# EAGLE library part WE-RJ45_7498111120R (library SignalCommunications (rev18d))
Order Code 7498111120R Design SMD xBase-T 10/100/1000 Base-T Ports 1x1 Application Standard Tab Position UP LED (Left-Right) YELLOW-GREEN EMI Fingers Yes Details see: http://katalog.we-online.de/en/pbs/WE-LAN_RJ45/7498111120R? Updated by Yingchun Shan 2016-08-23 2014 (C) Würth Elektronik
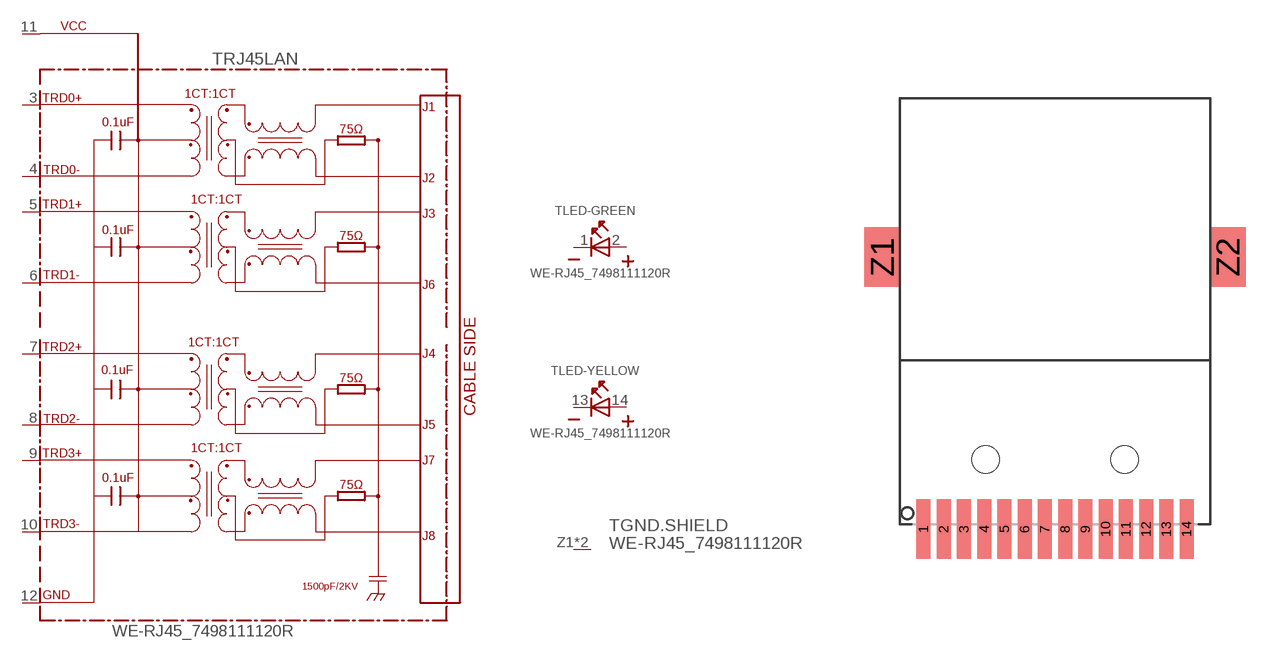
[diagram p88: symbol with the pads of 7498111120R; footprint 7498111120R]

Designator prefix T; gates RJ45LAN=7498111120R LED-GREEN=LED2PIN LED-YELLOW=LED2PIN GND.SHIELD=GNDPIN

## WE-RJ45_7498111120R (COMPANY-URL: http://www.we-online.de; CREATED-BY: Christin Zierenner; CREATED-DATE: AUG 2012; DATASHEET-URL: http://katalog.we-online.de/kataloge/eisos/media/pdf/7498111120R.pdf; MANUFACTURER: Würth Elektronik eiSos GmbH)  [7498111120R]
1  LED-GREEN:K  pas
2  LED-GREEN:A  pas
3  RJ45LAN:TRD0+
4  RJ45LAN:TRD0-
5  RJ45LAN:TRD1+
6  RJ45LAN:TRD1-
7  RJ45LAN:TRD2+
8  RJ45LAN:TRD2-
9  RJ45LAN:TRD3+
10  RJ45LAN:TRD3-
11  RJ45LAN:VCC  pwr
12  RJ45LAN:GND  pwr
13  LED-YELLOW:K  pas
14  LED-YELLOW:A  pas
Z1  GND.SHIELD:GND  pwr
Z2  GND.SHIELD:GND  pwr

## Footprint 7498111120R (pad centres in mm)
MAX HEIGHT=11.30mm PORTS----1X1 LED --Yes
smd 0.71 x 3: 1 -6.63,-3.5; 2 -5.61,-3.5; 3 -4.59,-3.5; 4 -3.57,-3.5; 5 -2.55,-3.5; 6 -1.53,-3.5; 7 -0.51,-3.5; 8 0.51,-3.5; 9 1.53,-3.5; 10 2.55,-3.5; 11 3.57,-3.5; 12 4.59,-3.5; 13 5.61,-3.5; 14 6.63,-3.5
smd 1.8 x 3: Z1 -8.71,10.2; Z2 8.71,10.2
hole 1.4 at -3.5,0
hole 1.4 at 3.5,0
